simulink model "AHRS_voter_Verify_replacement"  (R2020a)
settings: Solver=FixedStepDiscrete  StartTime=0.0  StopTime=10.0  FixedStep=0.01  RelTol=1e-3
undefined symbols (not defined in the file or in its folder): AHRS_voter, AHRS_voter_New, AHRS_voter_Original, Normal, sldvsubsys
libraries: simulink x2, sldvlib x1

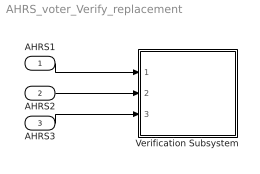
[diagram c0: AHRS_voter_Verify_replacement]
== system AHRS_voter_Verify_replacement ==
  AHRS1 : Inport  OutDataTypeStr=Bus: AHRS_Bus  PortDimensions=1  SampleTime=0.01
  AHRS2 : Inport  Port=2  OutDataTypeStr=Bus: AHRS_Bus  PortDimensions=1  SampleTime=0.01
  AHRS3 : Inport  Port=3  OutDataTypeStr=Bus: AHRS_Bus  PortDimensions=1  SampleTime=0.01
  Verification Subsystem : Subsystem  Tag=VerificationSubsystem  DisableCoverage=on  LoadFcn=sldvsubsys('check')  TreatAsAtomicUnit=on  SimViewingDevice=on  mask(VerificationSubsystem){}
      mask init:
      | sldvsubsys('maskInit');
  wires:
  AHRS1/1 -> Verification Subsystem/1(AHRS1)
  AHRS2/1 -> Verification Subsystem/2(AHRS2)
  AHRS3/1 -> Verification Subsystem/3(AHRS3)

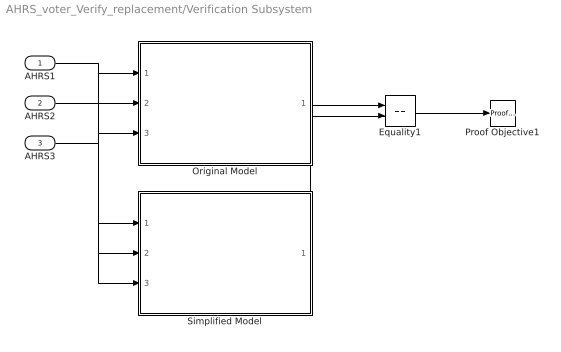
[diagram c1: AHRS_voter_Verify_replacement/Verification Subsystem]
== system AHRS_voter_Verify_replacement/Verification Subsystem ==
  AHRS1 : Inport  OutDataTypeStr=Bus: AHRS_Bus  PortDimensions=1  SampleTime=0.01
  AHRS2 : Inport  Port=2  OutDataTypeStr=Bus: AHRS_Bus  PortDimensions=1  SampleTime=0.01
  AHRS3 : Inport  Port=3  OutDataTypeStr=Bus: AHRS_Bus  PortDimensions=1  SampleTime=0.01
  Equality1 : RelationalOperator  Operator===  OutDataTypeStr=boolean  RndMeth=Simplest
  Original Model : Subsystem  TreatAsAtomicUnit=on  mask(Sldv ModelReference(Model name:AHRS_voter_Original) Replacement){ModelName=AHRS_voter_Original, ParameterArgumentNames=, ParameterArgumentValuesAsString=, SimulationMode=Normal}
      mask help: Replacement for the Model Reference block that references the model AHRS_voter_Original. If Model arguments are specified on the Model Reference block, then they will appear in the mask parameters.
  Proof Objective1 : sldvlib/Objectives and Constraints/Proof Objective  enabled=on  customAVTBlockType=Proof Objective  intervals=true  dispValues=on  outEnabled=off  enableStopSim=off
  Simplified Model : Subsystem  TreatAsAtomicUnit=on  mask(Sldv ModelReference(Model name:AHRS_voter_New) Replacement){ModelName=AHRS_voter_New, ParameterArgumentNames=, ParameterArgumentValuesAsString=, SimulationMode=Normal}
      mask help: Replacement for the Model Reference block that references the model AHRS_voter_New. If Model arguments are specified on the Model Reference block, then they will appear in the mask parameters.
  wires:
  AHRS1/1 -> Original Model/1(AHRS1), Simplified Model/1(AHRS1)
  AHRS2/1 -> Original Model/2(AHRS2), Simplified Model/2(AHRS2)
  AHRS3/1 -> Original Model/3(AHRS3), Simplified Model/3(AHRS3)
  Original Model/1(voted_fb) -> Equality1/1
  Simplified Model/1(voted_fb) -> Equality1/2
  Equality1/1 -> Proof Objective1/1

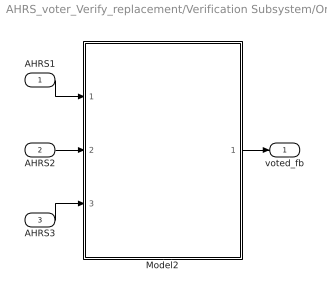
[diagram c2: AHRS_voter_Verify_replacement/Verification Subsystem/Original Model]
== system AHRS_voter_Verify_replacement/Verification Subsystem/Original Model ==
  AHRS1 : Inport  OutDataTypeStr=Bus: AHRS_Bus  PortDimensions=1  SampleTime=[0.01,0]
  AHRS2 : Inport  Port=2  OutDataTypeStr=Bus: AHRS_Bus  PortDimensions=1  SampleTime=[0.01,0]
  AHRS3 : Inport  Port=3  OutDataTypeStr=Bus: AHRS_Bus  PortDimensions=1  SampleTime=[0.01,0]
  Model2 : Subsystem  TreatAsAtomicUnit=on  mask(Sldv ModelReference(Model name:AHRS_voter) Replacement){ModelName=AHRS_voter, ParameterArgumentNames=, ParameterArgumentValuesAsString=, SimulationMode=Normal}
      mask help: Replacement for the Model Reference block that references the model AHRS_voter. If Model arguments are specified on the Model Reference block, then they will appear in the mask parameters.
  voted_fb : Outport  OutDataTypeStr=double  PortDimensions=5  SampleTime=[0.01,0]  VectorParamsAs1DForOutWhenUnconnected=off
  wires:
  Model2/1(voted_fb) -> voted_fb/1
  AHRS3/1 -> Model2/3(AHRS3)
  AHRS2/1 -> Model2/2(AHRS2)
  AHRS1/1 -> Model2/1(AHRS1)

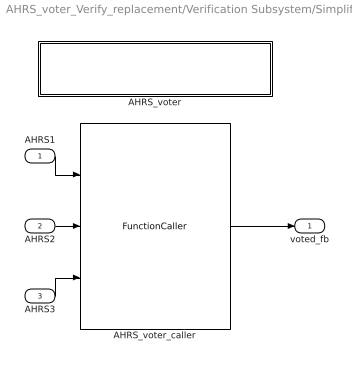
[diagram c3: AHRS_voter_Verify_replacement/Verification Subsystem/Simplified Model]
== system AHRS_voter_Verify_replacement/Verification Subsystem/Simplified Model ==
  AHRS1 : Inport  OutDataTypeStr=Bus: AHRS_Bus  PortDimensions=1  SampleTime=[0.01,0]
  AHRS2 : Inport  Port=2  OutDataTypeStr=Bus: AHRS_Bus  PortDimensions=1  SampleTime=[0.01,0]
  AHRS3 : Inport  Port=3  OutDataTypeStr=Bus: AHRS_Bus  PortDimensions=1  SampleTime=[0.01,0]
  AHRS_voter : Subsystem  TreatAsAtomicUnit=on
  AHRS_voter_caller : FunctionCaller  FunctionPrototype=voted_fb = AHRS_voter(AHRS1,AHRS2,AHRS3)  InputArgumentSpecifications=<Enter example>
  voted_fb : Outport  OutMin=-180  OutMax=180  OutDataTypeStr=double  PortDimensions=5  SampleTime=[0.01,0]  VectorParamsAs1DForOutWhenUnconnected=off
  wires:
  AHRS_voter_caller/1 -> voted_fb/1
  AHRS3/1 -> AHRS_voter_caller/3
  AHRS2/1 -> AHRS_voter_caller/2
  AHRS1/1 -> AHRS_voter_caller/1

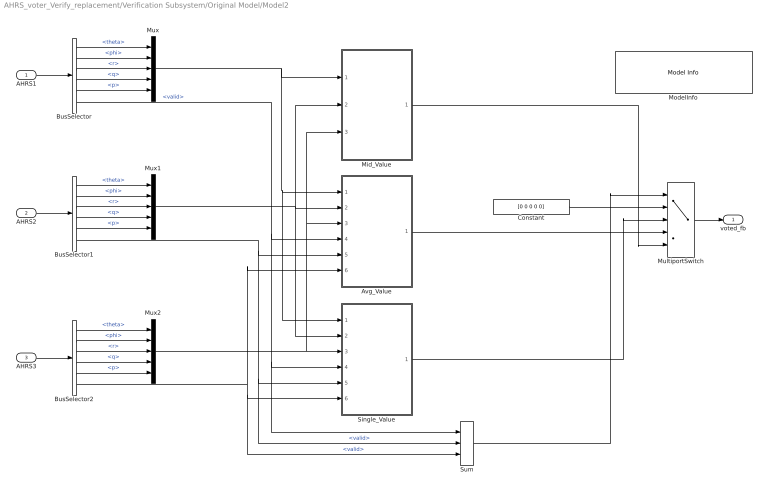
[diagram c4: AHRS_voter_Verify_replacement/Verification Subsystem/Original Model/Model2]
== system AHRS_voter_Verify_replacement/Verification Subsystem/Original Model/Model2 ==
  AHRS1 : Inport  OutDataTypeStr=Bus: AHRS_Bus  PortDimensions=1  SampleTime=[0.01,0]
  AHRS2 : Inport  Port=2  OutDataTypeStr=Bus: AHRS_Bus  PortDimensions=1  SampleTime=[0.01,0]
  AHRS3 : Inport  Port=3  OutDataTypeStr=Bus: AHRS_Bus  PortDimensions=1  SampleTime=[0.01,0]
  Avg_Value : Subsystem  TreatAsAtomicUnit=on  RTWFcnName=Avg_Value
  BusSelector : BusSelector  OutputSignals=theta,phi,r,q,p,valid
  BusSelector1 : BusSelector  OutputSignals=theta,phi,r,q,p,valid
  BusSelector2 : BusSelector  OutputSignals=theta,phi,r,q,p,valid
  Constant : Constant  Value=[0 0 0 0 0]
  Mid_Value : Subsystem  TreatAsAtomicUnit=on  RTWFcnName=Mid_Value
  ModelInfo : simulink/Model-Wide Utilities/Model Info  Frame=on  DisplayStringWithTags=|  HorizontalTextAlignment=Center  LeftAlignmentValue=0.5
      | Model Name: %<ModelName>
      | Model Version: %<ModelVersion>
      | Last Modified: %<LastModificationDate>
      | 
      | Copyright 2016 The MathWorks, Inc.
  MultiportSwitch : MultiPortSwitch  DataPortOrder=Zero-based contiguous  Inputs=4  DiagnosticForDefault=None  zeroidx=on
  Mux : Mux  Inputs=5
  Mux1 : Mux  Inputs=5
  Mux2 : Mux  Inputs=5
  Single_Value : Subsystem  TreatAsAtomicUnit=on  RTWFcnName=Single_Value
  Sum : Sum  Inputs=+++  OutDataTypeStr=uint32
  voted_fb : Outport  OutDataTypeStr=double  PortDimensions=5  SampleTime=[0.01,0]  VectorParamsAs1DForOutWhenUnconnected=off
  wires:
  BusSelector2/6 -> Single_Value/6(AHRS3_Valid), Sum/3, Avg_Value/6(AHRS3_Valid)  "<valid>"
  BusSelector2/5 -> Mux2/5  "<p>"
  BusSelector2/4 -> Mux2/4  "<q>"
  BusSelector2/3 -> Mux2/3  "<r>"
  BusSelector2/2 -> Mux2/2  "<phi>"
  BusSelector2/1 -> Mux2/1  "<theta>"
  AHRS3/1 -> BusSelector2/1
  Mux2/1 -> Mid_Value/3(AHRS3), Avg_Value/3(AHRS3), Single_Value/3(AHRS3)
  BusSelector1/6 -> Avg_Value/5(AHRS2_Valid), Sum/2, Single_Value/5(AHRS2_Valid)  "<valid>"
  Mux1/1 -> Single_Value/2(AHRS2), Mid_Value/2(AHRS2), Avg_Value/2(AHRS2)
  AHRS2/1 -> BusSelector1/1
  BusSelector1/1 -> Mux1/1  "<theta>"
  BusSelector1/2 -> Mux1/2  "<phi>"
  BusSelector1/3 -> Mux1/3  "<r>"
  BusSelector1/4 -> Mux1/4  "<q>"
  BusSelector1/5 -> Mux1/5  "<p>"
  Mux/1 -> Single_Value/1(AHRS1), Avg_Value/1(AHRS1), Mid_Value/1(AHRS1)
  BusSelector/5 -> Mux/5  "<p>"
  BusSelector/4 -> Mux/4  "<q>"
  BusSelector/3 -> Mux/3  "<r>"
  BusSelector/2 -> Mux/2  "<phi>"
  BusSelector/1 -> Mux/1  "<theta>"
  BusSelector/6 -> Single_Value/4(AHRS1_Valid), Sum/1, Avg_Value/4(AHRS1_Valid)  "<valid>"
  AHRS1/1 -> BusSelector/1
  Constant/1 -> MultiportSwitch/2
  Single_Value/1(Single_Value) -> MultiportSwitch/3
  Avg_Value/1(Avg_Value) -> MultiportSwitch/4
  Mid_Value/1(Mid_Value) -> MultiportSwitch/5
  Sum/1 -> MultiportSwitch/1
  MultiportSwitch/1 -> voted_fb/1

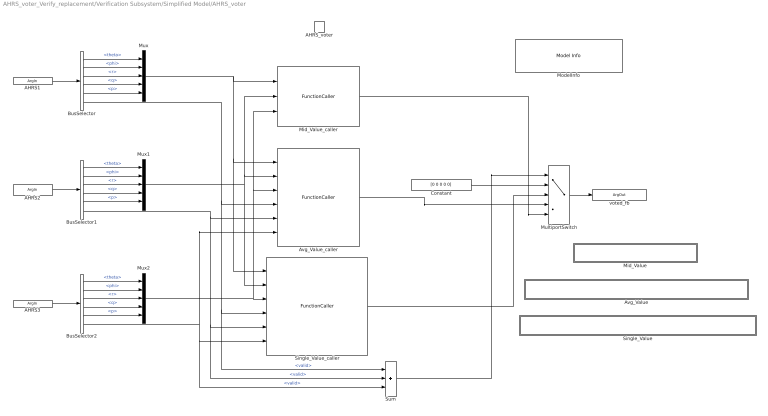
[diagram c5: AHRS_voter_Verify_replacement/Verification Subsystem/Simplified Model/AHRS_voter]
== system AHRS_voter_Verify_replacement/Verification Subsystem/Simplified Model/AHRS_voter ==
  AHRS_voter : TriggerPort  TriggerType=function-call  IsSimulinkFunction=on  FunctionName=AHRS_voter  FunctionVisibility=scoped  VariantControl=Variant  PortDimensions=1
  Avg_Value : Subsystem  TreatAsAtomicUnit=on  RTWFcnName=Avg_Value
  Avg_Value_caller : FunctionCaller  FunctionPrototype=Avg_Value = Avg_Value(AHRS1,AHRS2,AHRS3,AHRS1_Valid,AHRS2_Valid,AHRS3_Valid)
  BusSelector : BusSelector  OutputSignals=theta,phi,r,q,p,valid
  BusSelector1 : BusSelector  OutputSignals=theta,phi,r,q,p,valid
  BusSelector2 : BusSelector  OutputSignals=theta,phi,r,q,p,valid
  Constant : Constant  Value=[0 0 0 0 0]
  Mid_Value : Subsystem  TreatAsAtomicUnit=on  RTWFcnName=Mid_Value
  Mid_Value_caller : FunctionCaller  FunctionPrototype=Mid_Value = Mid_Value(AHRS1,AHRS2,AHRS3)
  ModelInfo : simulink/Model-Wide Utilities/Model Info  Frame=on  DisplayStringWithTags=|  HorizontalTextAlignment=Center  LeftAlignmentValue=0.5
      | Model Name: %<ModelName>
      | Model Version: %<ModelVersion>
      | Last Modified: %<LastModificationDate>
      | 
      | Copyright 2016 The MathWorks, Inc.
  MultiportSwitch : MultiPortSwitch  DataPortOrder=Zero-based contiguous  Inputs=4  DiagnosticForDefault=None  zeroidx=on
  Mux : Mux  Inputs=5
  Mux1 : Mux  Inputs=5
  Mux2 : Mux  Inputs=5
  Single_Value : Subsystem  TreatAsAtomicUnit=on  RTWFcnName=Single_Value
  Single_Value_caller : FunctionCaller  FunctionPrototype=Single_Value = Single_Value(AHRS1,AHRS2,AHRS3,AHRS1_Valid,AHRS2_Valid,AHRS3_Valid)
  Sum : Sum  Inputs=+++  OutDataTypeStr=uint32
  AHRS1 : ArgIn  OutDataTypeStr=Bus: AHRS_Bus  ArgumentName=AHRS1
  AHRS2 : ArgIn  Port=2  OutDataTypeStr=Bus: AHRS_Bus  ArgumentName=AHRS2
  AHRS3 : ArgIn  Port=3  OutDataTypeStr=Bus: AHRS_Bus  ArgumentName=AHRS3
  voted_fb : ArgOut  OutMin=-180  OutMax=180  PortDimensions=5  ArgumentName=voted_fb
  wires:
  BusSelector2/5 -> Mux2/5  "<p>"
  Mux2/1 -> Avg_Value_caller/3, Mid_Value_caller/3, Single_Value_caller/3
  BusSelector/4 -> Mux/4  "<q>"
  BusSelector2/1 -> Mux2/1  "<theta>"
  AHRS3/1 -> BusSelector2/1
  BusSelector/2 -> Mux/2  "<phi>"
  BusSelector2/2 -> Mux2/2  "<phi>"
  BusSelector2/3 -> Mux2/3  "<r>"
  BusSelector1/2 -> Mux1/2  "<phi>"
  Sum/1 -> MultiportSwitch/1
  BusSelector1/4 -> Mux1/4  "<q>"
  Constant/1 -> MultiportSwitch/2
  BusSelector2/4 -> Mux2/4  "<q>"
  BusSelector2/6 -> Sum/3, Single_Value_caller/6, Avg_Value_caller/6  "<valid>"
  BusSelector/6 -> Sum/1, Single_Value_caller/4, Avg_Value_caller/4  "<valid>"
  BusSelector1/3 -> Mux1/3  "<r>"
  BusSelector/1 -> Mux/1  "<theta>"
  Mux/1 -> Mid_Value_caller/1, Single_Value_caller/1, Avg_Value_caller/1
  AHRS2/1 -> BusSelector1/1
  BusSelector/3 -> Mux/3  "<r>"
  Single_Value_caller/1 -> MultiportSwitch/3
  BusSelector1/1 -> Mux1/1  "<theta>"
  BusSelector1/5 -> Mux1/5  "<p>"
  Mux1/1 -> Single_Value_caller/2, Avg_Value_caller/2, Mid_Value_caller/2
  BusSelector/5 -> Mux/5  "<p>"
  MultiportSwitch/1 -> voted_fb/1
  AHRS1/1 -> BusSelector/1
  Mid_Value_caller/1 -> MultiportSwitch/5
  Avg_Value_caller/1 -> MultiportSwitch/4
  BusSelector1/6 -> Sum/2, Single_Value_caller/5, Avg_Value_caller/5  "<valid>"

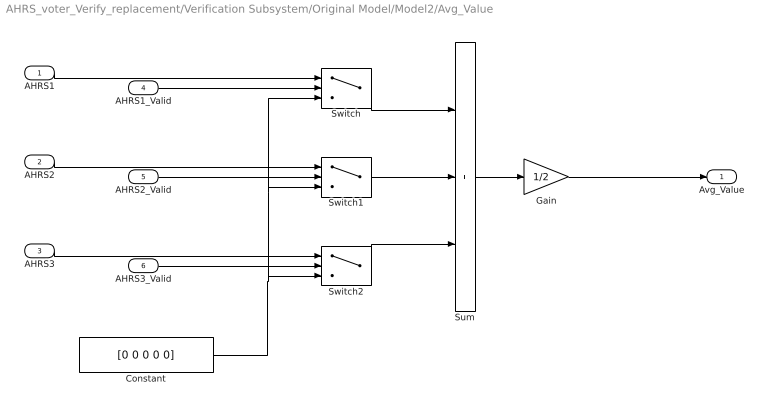
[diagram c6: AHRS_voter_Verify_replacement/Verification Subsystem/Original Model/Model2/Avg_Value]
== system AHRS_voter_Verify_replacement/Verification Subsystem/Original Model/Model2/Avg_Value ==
  AHRS1 : Inport
  AHRS2 : Inport  Port=2
  AHRS3 : Inport  Port=3
  AHRS1_Valid : Inport  Port=4  OutDataTypeStr=boolean  PortDimensions=1
  AHRS2_Valid : Inport  Port=5  OutDataTypeStr=boolean  PortDimensions=1
  AHRS3_Valid : Inport  Port=6  OutDataTypeStr=boolean  PortDimensions=1
  Constant : Constant  Value=[0 0 0 0 0]
  Gain : Gain  Gain=1/2
  Sum : Sum  Inputs=+++
  Switch : Switch  Criteria=u2 ~= 0
  Switch1 : Switch  Criteria=u2 ~= 0
  Switch2 : Switch  Criteria=u2 ~= 0
  Avg_Value : Outport  VectorParamsAs1DForOutWhenUnconnected=off
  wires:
  Gain/1 -> Avg_Value/1
  Sum/1 -> Gain/1
  AHRS1_Valid/1 -> Switch/2
  AHRS1/1 -> Switch/1
  Switch/1 -> Sum/1
  Switch1/1 -> Sum/2
  Switch2/1 -> Sum/3
  AHRS2_Valid/1 -> Switch1/2
  AHRS3_Valid/1 -> Switch2/2
  AHRS2/1 -> Switch1/1
  AHRS3/1 -> Switch2/1
  Constant/1 -> Switch/3, Switch1/3, Switch2/3

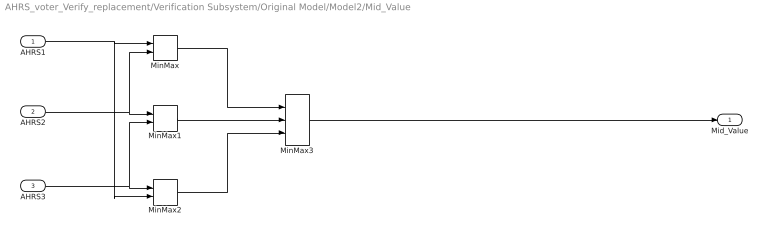
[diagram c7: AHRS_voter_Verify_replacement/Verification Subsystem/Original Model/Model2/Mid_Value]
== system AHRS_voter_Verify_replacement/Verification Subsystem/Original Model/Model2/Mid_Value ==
  AHRS1 : Inport
  AHRS2 : Inport  Port=2
  AHRS3 : Inport  Port=3
  MinMax : MinMax  Inputs=2
  MinMax1 : MinMax  Inputs=2
  MinMax2 : MinMax  Inputs=2
  MinMax3 : MinMax  Function=max  Inputs=3
  Mid_Value : Outport  VectorParamsAs1DForOutWhenUnconnected=off
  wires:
  AHRS1/1 -> MinMax2/2, MinMax/1
  AHRS3/1 -> MinMax1/2, MinMax2/1
  AHRS2/1 -> MinMax/2, MinMax1/1
  MinMax1/1 -> MinMax3/2
  MinMax/1 -> MinMax3/1
  MinMax2/1 -> MinMax3/3
  MinMax3/1 -> Mid_Value/1

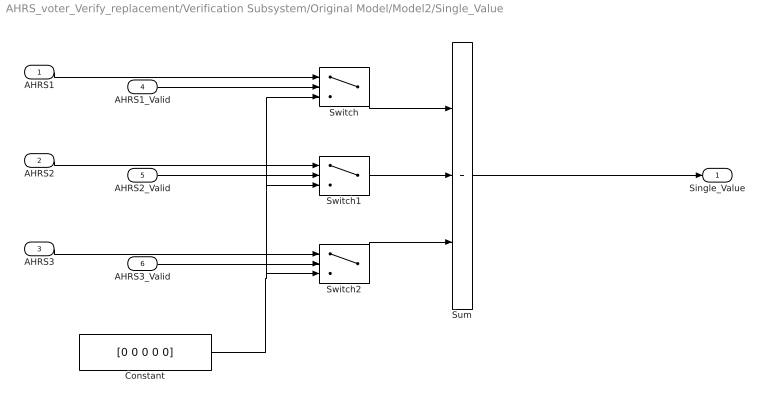
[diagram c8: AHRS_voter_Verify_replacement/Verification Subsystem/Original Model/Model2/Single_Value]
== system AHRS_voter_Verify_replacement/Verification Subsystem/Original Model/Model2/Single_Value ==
  AHRS1 : Inport
  AHRS2 : Inport  Port=2
  AHRS3 : Inport  Port=3
  AHRS1_Valid : Inport  Port=4  OutDataTypeStr=boolean  PortDimensions=1
  AHRS2_Valid : Inport  Port=5  OutDataTypeStr=boolean  PortDimensions=1
  AHRS3_Valid : Inport  Port=6  OutDataTypeStr=boolean  PortDimensions=1
  Constant : Constant  Value=[0 0 0 0 0]
  Sum : Sum  Inputs=+++
  Switch : Switch  Criteria=u2 ~= 0
  Switch1 : Switch  Criteria=u2 ~= 0
  Switch2 : Switch  Criteria=u2 ~= 0
  Single_Value : Outport  VectorParamsAs1DForOutWhenUnconnected=off
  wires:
  Constant/1 -> Switch2/3, Switch1/3, Switch/3
  AHRS3/1 -> Switch2/1
  AHRS2/1 -> Switch1/1
  AHRS3_Valid/1 -> Switch2/2
  AHRS2_Valid/1 -> Switch1/2
  Switch2/1 -> Sum/3
  Switch1/1 -> Sum/2
  Switch/1 -> Sum/1
  AHRS1/1 -> Switch/1
  AHRS1_Valid/1 -> Switch/2
  Sum/1 -> Single_Value/1

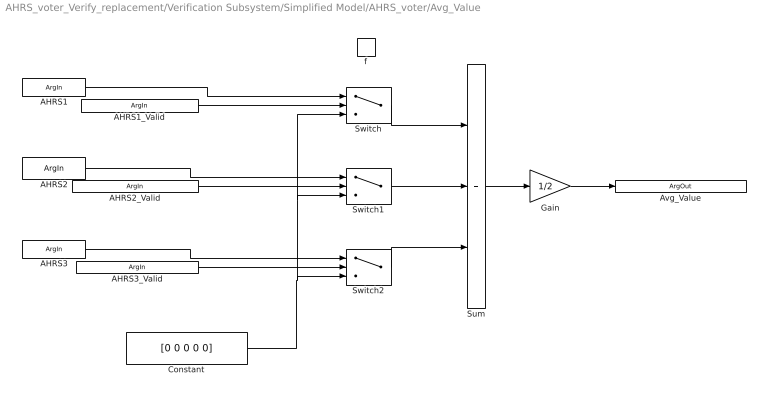
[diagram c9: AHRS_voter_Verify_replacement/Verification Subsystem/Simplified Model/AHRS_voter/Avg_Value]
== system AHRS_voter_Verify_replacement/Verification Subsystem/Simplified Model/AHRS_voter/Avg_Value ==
  f : TriggerPort  TriggerType=function-call  IsSimulinkFunction=on  FunctionName=Avg_Value  FunctionVisibility=scoped  VariantControl=Variant  PortDimensions=1
  Constant : Constant  Value=[0 0 0 0 0]
  Gain : Gain  Gain=1/2
  Sum : Sum  Inputs=+++
  Switch : Switch  Criteria=u2 ~= 0
  Switch1 : Switch  Criteria=u2 ~= 0
  Switch2 : Switch  Criteria=u2 ~= 0
  AHRS1 : ArgIn  PortDimensions=5  ArgumentName=AHRS1
  AHRS2 : ArgIn  Port=2  PortDimensions=5  ArgumentName=AHRS2
  AHRS3 : ArgIn  Port=3  PortDimensions=5  ArgumentName=AHRS3
  AHRS1_Valid : ArgIn  Port=4  OutDataTypeStr=boolean  ArgumentName=AHRS1_Valid
  AHRS2_Valid : ArgIn  Port=5  OutDataTypeStr=boolean  ArgumentName=AHRS2_Valid
  AHRS3_Valid : ArgIn  Port=6  OutDataTypeStr=boolean  ArgumentName=AHRS3_Valid
  Avg_Value : ArgOut  PortDimensions=5  ArgumentName=Avg_Value
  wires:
  Gain/1 -> Avg_Value/1
  Sum/1 -> Gain/1
  AHRS1_Valid/1 -> Switch/2
  AHRS1/1 -> Switch/1
  Switch/1 -> Sum/1
  Switch1/1 -> Sum/2
  Switch2/1 -> Sum/3
  AHRS2_Valid/1 -> Switch1/2
  AHRS3_Valid/1 -> Switch2/2
  AHRS2/1 -> Switch1/1
  AHRS3/1 -> Switch2/1
  Constant/1 -> Switch/3, Switch1/3, Switch2/3

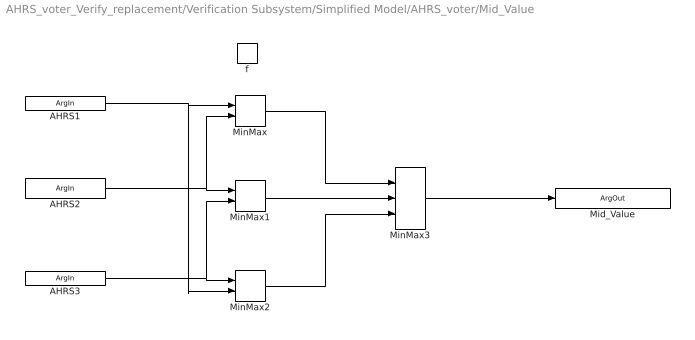
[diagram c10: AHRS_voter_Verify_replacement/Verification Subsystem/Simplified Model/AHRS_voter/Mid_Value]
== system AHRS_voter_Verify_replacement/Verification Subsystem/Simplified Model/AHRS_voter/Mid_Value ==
  f : TriggerPort  TriggerType=function-call  IsSimulinkFunction=on  FunctionName=Mid_Value  FunctionVisibility=scoped  VariantControl=Variant  PortDimensions=1
  MinMax : MinMax  Inputs=2
  MinMax1 : MinMax  Inputs=2
  MinMax2 : MinMax  Inputs=2
  MinMax3 : MinMax  Function=max  Inputs=3
  AHRS1 : ArgIn  PortDimensions=5  ArgumentName=AHRS1
  AHRS2 : ArgIn  Port=2  PortDimensions=5  ArgumentName=AHRS2
  AHRS3 : ArgIn  Port=3  PortDimensions=5  ArgumentName=AHRS3
  Mid_Value : ArgOut  PortDimensions=5  ArgumentName=Mid_Value
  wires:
  AHRS1/1 -> MinMax2/2, MinMax/1
  AHRS3/1 -> MinMax1/2, MinMax2/1
  AHRS2/1 -> MinMax/2, MinMax1/1
  MinMax1/1 -> MinMax3/2
  MinMax/1 -> MinMax3/1
  MinMax2/1 -> MinMax3/3
  MinMax3/1 -> Mid_Value/1

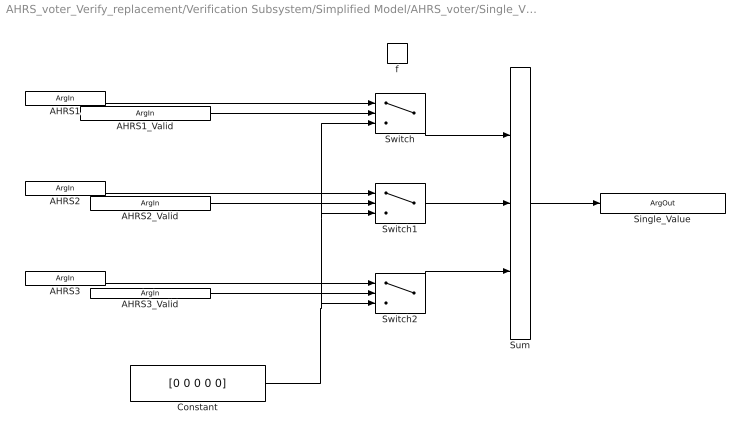
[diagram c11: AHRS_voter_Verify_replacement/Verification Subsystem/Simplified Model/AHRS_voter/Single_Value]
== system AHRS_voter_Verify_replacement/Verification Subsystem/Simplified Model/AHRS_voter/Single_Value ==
  f : TriggerPort  TriggerType=function-call  IsSimulinkFunction=on  FunctionName=Single_Value  FunctionVisibility=scoped  VariantControl=Variant  PortDimensions=1
  Constant : Constant  Value=[0 0 0 0 0]
  Sum : Sum  Inputs=+++
  Switch : Switch  Criteria=u2 ~= 0
  Switch1 : Switch  Criteria=u2 ~= 0
  Switch2 : Switch  Criteria=u2 ~= 0
  AHRS1 : ArgIn  PortDimensions=5  ArgumentName=AHRS1
  AHRS2 : ArgIn  Port=2  PortDimensions=5  ArgumentName=AHRS2
  AHRS3 : ArgIn  Port=3  PortDimensions=5  ArgumentName=AHRS3
  AHRS1_Valid : ArgIn  Port=4  OutDataTypeStr=boolean  ArgumentName=AHRS1_Valid
  AHRS2_Valid : ArgIn  Port=5  OutDataTypeStr=boolean  ArgumentName=AHRS2_Valid
  AHRS3_Valid : ArgIn  Port=6  OutDataTypeStr=boolean  ArgumentName=AHRS3_Valid
  Single_Value : ArgOut  PortDimensions=5  ArgumentName=Single_Value
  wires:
  Constant/1 -> Switch2/3, Switch1/3, Switch/3
  AHRS3/1 -> Switch2/1
  AHRS2/1 -> Switch1/1
  AHRS3_Valid/1 -> Switch2/2
  AHRS2_Valid/1 -> Switch1/2
  Switch2/1 -> Sum/3
  Switch1/1 -> Sum/2
  Switch/1 -> Sum/1
  AHRS1/1 -> Switch/1
  AHRS1_Valid/1 -> Switch/2
  Sum/1 -> Single_Value/1
